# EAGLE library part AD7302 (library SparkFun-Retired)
8-bit parallel input 2-output DAC Retired: IC-09157
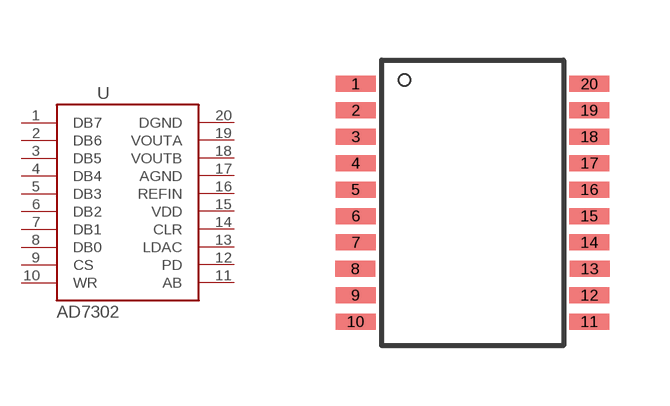
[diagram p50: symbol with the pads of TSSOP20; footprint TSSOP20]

Designator prefix -

## AD7302SMD  [TSSOP20]
1  DB7
2  DB6
3  DB5
4  DB4
5  DB3
6  DB2
7  DB1
8  DB0
9  CS
10  WR
11  AB
12  PD
13  LDAC
14  CLR
15  VDD
16  REFIN
17  AGND
18  VOUTB
19  VOUTA
20  DGND

## Footprint TSSOP20 (pad centres in mm)
smd 1 x 0.4: 1 -2.937,2.693; 2 -2.937,2.032; 3 -2.937,1.372; 4 -2.937,0.712; 5 -2.937,0.051; 6 -2.937,-0.609; 7 -2.937,-1.27; 8 -2.943,-1.93; 9 -2.937,-2.59; 10 -2.937,-3.251; 11 2.905,-3.251; 12 2.905,-2.59; 13 2.911,-1.93; 14 2.905,-1.27; 15 2.905,-0.609; 16 2.905,0.051; 17 2.905,0.712; 18 2.905,1.372; 19 2.905,2.032; 20 2.905,2.693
